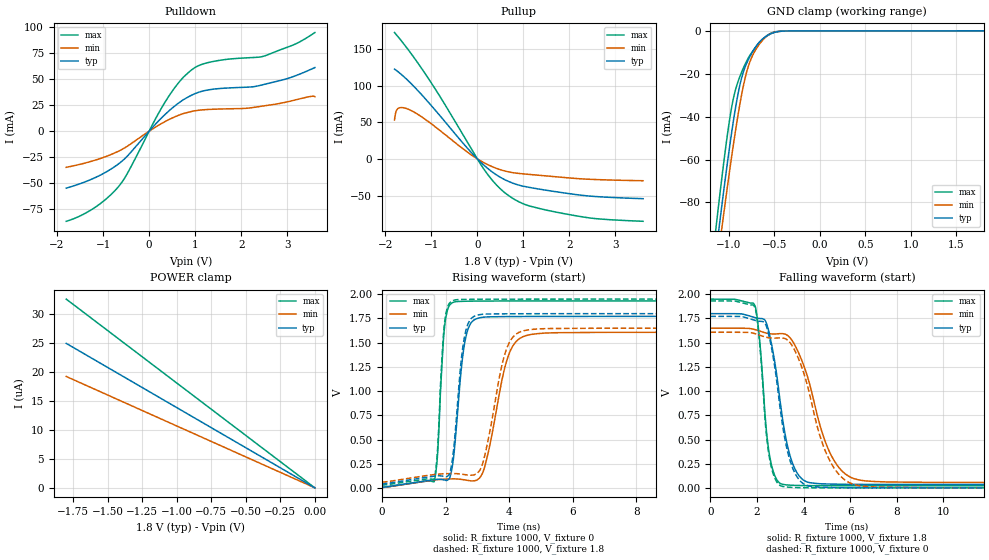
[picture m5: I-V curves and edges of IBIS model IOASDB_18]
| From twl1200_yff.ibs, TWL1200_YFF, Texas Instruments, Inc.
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[Model]   IOASDB_18
Model_type  I/O
Vinl=0.63
Vinh=1.17
Enable   Active-Low
Vref =   1.8
Rref =   1M
Cref =   15p
Vmeas =   0.9
| variable   typ   min   max
C_comp   4.20pF   3.56pF   5.01pF
| C_pullup   6.61pF   4.03pF   7.91pF
| C_pulldown   5.69pF   4.71pF   6.59pF
| C_tri-state   4.20pF   3.56pF   5.01pF
[Temperature Range]   40   100   -40
| Ambient temperature   25   85   -40
[Voltage range]   1.8   1.65   1.95
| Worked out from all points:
|   slope of the pulldown table from 0 to 0.27 V, typ, clamps not added: 21.1 ohm
|   slope of the pullup table from 0 to 0.27 V, typ, clamps not added: 17.7 ohm
|   GND clamp passes 1 mA (typ) near -0.51 V on its own axis
|   rising waveform, R_fixture 1000, V_fixture 0: 20-80 % time 299ps typ, 589ps min, 181ps max; typ from 0.001 V to 1.77 V
|   falling waveform, R_fixture 1000, V_fixture 1.8: 20-80 % time 701ps typ, 1.21ns min, 395ps max; typ from 1.8 V to 0.036 V
|   rising waveform, R_fixture 1000, V_fixture 1.8: 20-80 % time 291ps typ, 561ps min, 180ps max; typ from 0.036 V to 1.8 V
|   falling waveform, R_fixture 1000, V_fixture 0: 20-80 % time 689ps typ, 1.18ns min, 390ps max; typ from 1.77 V to 0.001 V
[GND Clamp]
| IOASDB_18
|   Voltage   I(typ)   I(min)   I(max)
-1.8V     -350.5mA   -347.3mA   -356.7mA
-1.14V    -104.2mA   -113.8mA   -92.69mA
-1.125V   -99.04mA   -108.9mA   -87.15mA
-1.095V   -88.75mA   -99.02mA   -76.27mA
-1.065V   -78.65mA   -89.31mA   -65.72mA
-955mV    -44.37mA   -55.5mA    -33.26mA
-900mV    -30.34mA   -40.32mA   -24.22mA
-850mV    -21.02mA   -28.36mA   -18.63mA
-795mV    -14.55mA   -18.29mA   -13.61mA
-735mV    -9.659mA   -11.41mA   -9.515mA
-550mV    -1.676mA   -1.638mA   -1.44mA
1.8V      421.1pA    1.603uA    -2.71uA
[POWER Clamp]
| IOASDB_18
|   Voltage   I(typ)   I(min)   I(max)
-1.8V     24.89uA    19.19uA    32.51uA
-170mV    2.352uA    1.816uA    3.071uA
-60mV     832.8nA    647.8nA    1.086uA
0V        0A         0A         0A
[Pulldown]
| IOASDB_18
|   Voltage   I(typ)   I(min)   I(max)
-1.8V     -54.74mA   -34.76mA   -86.6mA
-1.19V    -45mA      -28.11mA   -73.69mA
-665mV    -31.45mA   -19.23mA   -53.3mA
-460mV    -23.33mA   -14.08mA   -39.58mA
125mV     6.108mA    3.541mA    10.72mA
370mV     17.01mA    9.764mA    29.59mA
670mV     27.97mA    15.75mA    48.14mA
930mV     34.72mA    19.02mA    59.13mA
1.42V     40.49mA    21.11mA    67.21mA
2.495V    44.89mA    24.29mA    72.1mA
3.18V     53.24mA    30.04mA    83.79mA
3.6V      61.09mA    33.19mA    94.73mA
[Pullup]
| IOASDB_18
|   Voltage   I(typ)   I(min)   I(max)
-1.8V     122.6mA    53.1mA     172.5mA
-1.765V   121mA      64.88mA    169.9mA
-1.72V    118.8mA    68.89mA    166.5mA
-1.47V    104.7mA    66.97mA    146.4mA
-860mV    62.51mA    41.12mA    90mA
135mV     -8.14mA    -4.929mA   -13.33mA
385mV     -20.58mA   -12.22mA   -33.51mA
635mV     -29.58mA   -17.11mA   -48.08mA
1.055V    -38mA      -20.79mA   -62.71mA
1.7V      -44.77mA   -24.38mA   -72.54mA
2.52V     -51.17mA   -28.06mA   -81.23mA
3.6V      -54.35mA   -29.83mA   -85.21mA
[Ramp]
| IOASDB_18
| variable   typ   min   max
dV/dt_r   1.06/3.09E-10   0.96/5.94E-10   1.16/1.88E-10
dV/dt_f   1.06/7.02E-10   0.96/1.21E-09   1.16/4.02E-10
R_load = 1000
[Rising Waveform]
| IOASDB_18
R_fixture =   1000
C_fixture =   0
L_fixture =   0
V_fixture =   0
V_fixture_min = 0
V_fixture_max = 0
|   Time   V(typ)   V(min)   V(max)
0s        1.303mV    1.445mV    1.209mV
1.64ns    85.51mV    82.16mV    63.25mV
1.74ns    89.58mV    85.53mV    311.5mV
1.955ns   82.85mV    91mV       1.619V
2.125ns   100mV      93.51mV    1.887V
2.625ns   1.538V     82mV       1.928V
3.185ns   1.763V     169.4mV    1.93V
4.125ns   1.77V      1.471V     1.931V
5.44ns    1.772V     1.603V     1.931V
239.8ns   1.772V     1.608V     1.931V
[Falling Waveform]
| IOASDB_18
R_fixture =   1000
C_fixture =   0
L_fixture =   0
V_fixture =   1.8
V_fixture_min = 1.65
V_fixture_max = 1.95
|   Time   V(typ)   V(min)   V(max)
0s        1.8V       1.65V      1.95V
1.93ns    1.759V     1.635V     1.874V
2.14ns    1.75V      1.619V     1.464V
2.36ns    1.726V     1.602V     721.3mV
2.79ns    1.264V     1.59V      114.6mV
3.24ns    515.8mV    1.585V     32.6mV
3.685ns   171mV      1.448V     26.45mV
5.405ns   39.26mV    247.9mV    23.12mV
7.625ns   36.66mV    61.8mV     22.95mV
239.8ns   36.42mV    56.3mV     22.94mV
[Rising Waveform]
| IOASDB_18
R_fixture =   1000
C_fixture =   0
L_fixture =   0
V_fixture =   1.8
V_fixture_min = 1.65
V_fixture_max = 1.95
|   Time   V(typ)   V(min)   V(max)
0s        36.42mV    56.3mV     22.94mV
1.64ns    121.6mV    138.4mV    88.26mV
1.995ns   117.2mV    147.3mV    1.774V
2.22ns    305.8mV    149.1mV    1.933V
2.485ns   1.296V     143.4mV    1.946V
2.715ns   1.702V     133.3mV    1.948V
3.16ns    1.793V     245.6mV    1.949V
4.035ns   1.799V     1.519V     1.95V
5.225ns   1.8V       1.646V     1.95V
239.8ns   1.8V       1.65V      1.95V
[Falling Waveform]
| IOASDB_18
R_fixture =   1000
C_fixture =   0
L_fixture =   0
V_fixture =   0
V_fixture_min = 0
V_fixture_max = 0
|   Time   V(typ)   V(min)   V(max)
0s        1.772V     1.608V     1.931V
1.91ns    1.732V     1.594V     1.865V
2.115ns   1.722V     1.578V     1.5V
2.36ns    1.695V     1.559V     675.1mV
2.79ns    1.209V     1.548V     89.66mV
3.215ns   486.5mV    1.542V     11.15mV
3.665ns   137.1mV    1.401V     4.742mV
5.31ns    4.362mV    205.6mV    1.413mV
7.47ns    1.557mV    7.034mV    1.221mV
239.8ns   1.303mV    1.445mV    1.209mV
